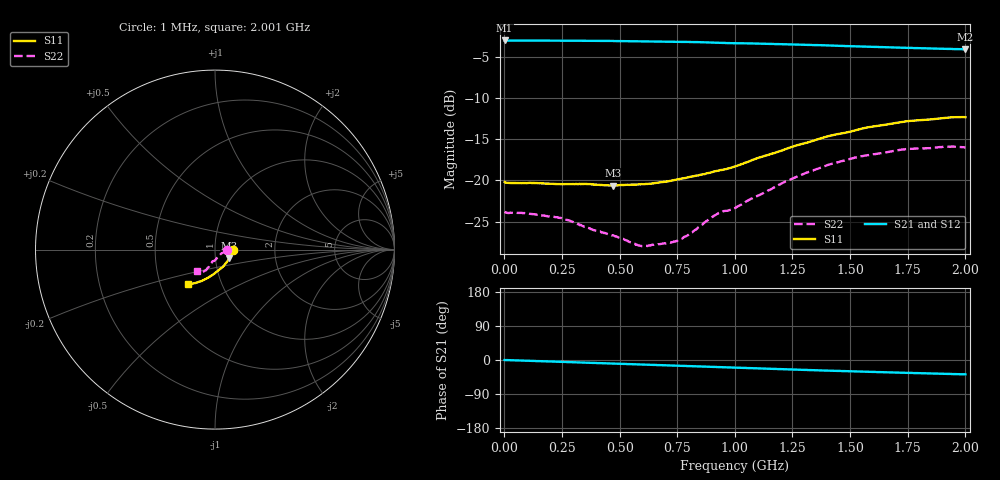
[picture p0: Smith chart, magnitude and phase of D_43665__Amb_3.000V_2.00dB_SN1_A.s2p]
! device id: 43665_
! dir: \\malibu\benchdata\1_engineers\tn_data\43665_75ohm\new\sparar\43665_\amb\3p000v\2p00db
! Serial: 1
! Insertion: A
! Temp: Amb
! VDD: 3.000V
! Attenuation Step: 2.00dB
! IDD: 1.452756e+00mA
! FILE NAME
! DATE 03-27-2009 08:33:51
! CORRECTED  DATA
#  Hz  S  RI  R  75
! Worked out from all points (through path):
!   401 points, 1 MHz to 2.001 GHz, reference 75 ohm
!   highest |S21| = -3.01 dB at 1 MHz (marker M1); lowest = -4.1 dB at 2.001 GHz (marker M2)
!   group delay of S21, straight-line fit = 53.7 ps
!   lowest |S11| = -20.6 dB at 471 MHz (marker M3), VSWR 1.21, Z = 87.6 - j8.37 ohm
!   |S11| at or under -10 dB: start of sweep to end of sweep
!   |S22| runs from -28.0 to -15.9 dB; largest |S21 - S12| = 0.0034
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1000000  0.0977 -0.00151  0.7071 -0.0011  0.7072 -0.00103  0.0645 -0.000677
9.6e7  0.0958 -0.00856  0.7056 -0.0234  0.7058 -0.0235  0.0632 -0.00134
2.36e8  0.0924 -0.0218  0.7027 -0.0572  0.7029 -0.0575  0.059 -0.00515
2.86e8  0.0909 -0.0271  0.7012 -0.0693  0.7015 -0.0696  0.0564 -0.00606
3.36e8  0.0896 -0.0324  0.6992 -0.0815  0.6993 -0.0817  0.0526 -0.00781
4.71e8  0.0801 -0.0474  0.6925 -0.1141  0.6925 -0.1146  0.0437 -0.0157
5.91e8  0.0703 -0.0631  0.6841 -0.1429  0.6839 -0.1433  0.0319 -0.0242
6.71e8  0.0619 -0.0748  0.6781 -0.1621  0.6778 -0.1623  0.0252 -0.0322
7.31e8  0.0547 -0.0837  0.6725 -0.1765  0.6725 -0.1768  0.0193 -0.0375
7.61e8  0.0508 -0.0884  0.6695 -0.1838  0.6694 -0.1839  0.016 -0.0408
8.06e8  0.0445 -0.0953  0.6646 -0.1947  0.6644 -0.1948  0.0108 -0.0463
9.21e8  0.0236 -0.1116  0.648 -0.2208  0.6482 -0.2206  -0.00341 -0.0622
1.001e9  0.0124 -0.1209  0.6391 -0.2337  0.6394 -0.2337  -0.0151 -0.0663
1.211e9  -0.0287 -0.1504  0.6121 -0.2771  0.6129 -0.2776  -0.0315 -0.0919
1.336e9  -0.0541 -0.1645  0.5927 -0.2985  0.5935 -0.2993  -0.044 -0.1058
1.406e9  -0.0688 -0.1721  0.5814 -0.3109  0.5822 -0.3123  -0.0491 -0.1142
1.511e9  -0.0885 -0.1785  0.565 -0.3254  0.5652 -0.327  -0.0618 -0.1215
1.586e9  -0.1021 -0.1847  0.5535 -0.3361  0.5535 -0.3385  -0.0676 -0.1259
1.671e9  -0.1152 -0.1872  0.5407 -0.3469  0.5396 -0.3488  -0.0765 -0.1281
1.741e9  -0.1257 -0.1901  0.53 -0.3554  0.5291 -0.3575  -0.0826 -0.1308
1.911e9  -0.1444 -0.1911  0.5056 -0.3742  0.5042 -0.3744  -0.0977 -0.1265
2.001e9  -0.1506 -0.1895  0.4936 -0.3836  0.4904 -0.3848  -0.1025 -0.121
